VAR_GLOBAL CONSTANT
	
	cOversamples 	: UDINT 	:= 10;		// number of oversamples
	cBufferLength	: UDINT		:= 2048;
	cWindowLength   : UDINT     := 2 * cBufferLength;
	cFFTLength		: UDINT		:= 4096;	// length of FFT and IFFT		 	
	cFFTResult 		: UDINT 	:= cFFTLength/2+1;
		
END_VAR
